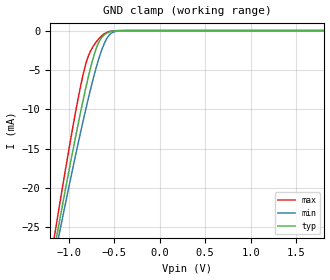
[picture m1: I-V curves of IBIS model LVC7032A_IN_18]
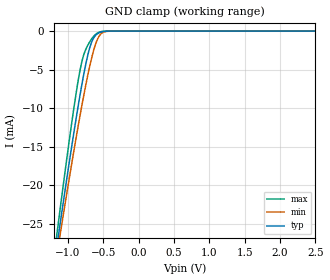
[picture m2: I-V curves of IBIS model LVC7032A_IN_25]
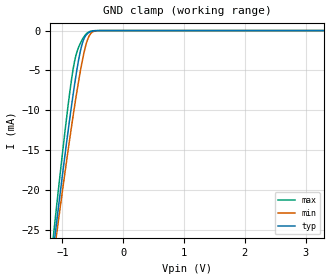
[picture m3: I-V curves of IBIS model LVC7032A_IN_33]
| TEXAS INSTRUMENTS INCORPORATED
| IBIS Model of SN74LVC7032A
| This file provides unique models under the [Model Selector] for each Vcc.
| For operation at a specific Vcc, select the appropriate model after each
| [Model Selector] keyword.
[IBIS Ver]   3.2
[Comment char]  |_char
[File Name]   sn74lvc7032aq1.ibs
[File Rev]   1
[Date]   October 2, 2023
[Source]   Data created from TI-SPICE simulations.
[Disclaimer] Property of Texas Instruments Incorporated.  Unauthorized
   reproduction and/or distribution is strictly prohibited.
   This product is protected under copyright law.
   Created  2023, (C) Copyright  2023, Texas Instruments
   Incorporated, All Rights Reserved
   UNLESS THERE IS A SIGNED, WRITTEN AGREEMENT TO THE
   CONTRARY, TEXAS INSTRUMENTS (TI) IS PROVIDING THE IBIS
   MODELS  AND WITHOUT ANY WARRANTY, EXPRESSED OR
   IMPLIED.  TI assumes no liability for:
   1) the accuracy of the IBIS models provided to your
   company;
   2) the proper functioning of these IBIS Models in your
   design or for any resulting applications; or
   3) infringement of patents, copyrights or intellectual
   property rights resulting from your use of these IBIS
   models.
   TI provides IBIS Models as a service to our customers.
   You and your company shall not distribute, sell or give
   these models to anyone else without prior written
   permission from TI.
   TI reserves the right to make changes to our products or
   to discontinue any semiconductor product or service
   without notice, and advises our customers to obtain the
   latest version of relevant information to verify, before
   placing orders, that the information being relied on is
   current.
   Please be aware that your receipt and use of the IBIS
   information provided shall serve as acceptance of these
   terms and conditions.  If you do not accept these terms,
   you should return or destroy the IBIS models and any
   other accompanying information immediately.
| Component LVC7032A_BQA 14-pin WQFN
[Component]   LVC7032A_BQA
[Manufacturer]   TI
[Package]   |14 WQFN - BQA package
|   typ   min   max
R_pkg   0.05   0.04   0.06
L_pkg   1.0nH   0.8nH   1.2nH
C_pkg   0.2pF   0.16pF   0.24pF
[Pin]   signal_name   model_name   R_pin   L_pin   C_pin
1   1A   LVC7032A_IN   NA   NA   NA
2   1B   LVC7032A_IN   NA   NA   NA
3   1Y   LVC7032A_OUT   NA   NA   NA
4   2A   LVC7032A_IN   NA   NA   NA
5   2B   LVC7032A_IN   NA   NA   NA
6   2Y   LVC7032A_OUT   NA   NA   NA
7   GND   GND   NA   NA   NA
8   3Y   LVC7032A_OUT   NA   NA   NA
9   3A   LVC7032A_IN   NA   NA   NA
10   3B   LVC7032A_IN   NA   NA   NA
11   4Y   LVC7032A_OUT   NA   NA   NA
12   4A   LVC7032A_IN   NA   NA   NA
13   4B   LVC7032A_IN   NA   NA   NA
14   VCC   POWER   NA   NA   NA
[Model Selector]   LVC7032A_IN
LVC7032A_IN_18   1.8 volt Vcc
LVC7032A_IN_25   2.5 volt Vcc
LVC7032A_IN_33   3.3 volt Vcc
| Model LVC7032A_OUT
[Model Selector]   LVC7032A_OUT
LVC7032A_OUT_18   1.8 volt Vcc
LVC7032A_OUT_25   2.5 volt Vcc
LVC7032A_OUT_33   3.3 volt Vcc
| Models and submodels in the file (6): LVC7032A_IN_18 (Input), LVC7032A_IN_25 (Input), LVC7032A_IN_33 (Input), LVC7032A_OUT_18 (Output), LVC7032A_OUT_25 (Output), LVC7032A_OUT_33 (Output)
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[Model]   LVC7032A_IN_18
Model_type  Input
Vinl=0.4
Vinh=0.85
| variable   typ   min   max
C_comp   2.66pF   2.19pF   3.17pF
[Temperature Range]   40   100   -40
| Ambient temperature   25   85   -40
[Voltage range]   1.8   1.65   1.95
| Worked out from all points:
|   GND clamp passes 1 mA (typ) near -0.64 V on its own axis
[GND Clamp]
| LVC7032A_IN_18
|   Voltage   I(typ)   I(min)   I(max)
-5.5V     -338.9mA   -314.3mA   -369mA
-1.16V    -28.09mA   -29.24mA   -26.56mA
-1.12V    -25.56mA   -26.92mA   -23.71mA
-1.085V   -23.36mA   -24.91mA   -21.25mA
-925mV    -13.65mA   -15.98mA   -10.52mA
-820mV    -7.797mA   -10.48mA   -4.654mA
-770mV    -5.293mA   -8.026mA   -2.891mA
-695mV    -2.253mA   -4.666mA   -1.432mA
-600mV    -473.7uA   -1.449mA   -358.4uA
-535mV    -136.2uA   -379.8uA   -78.5uA
-445mV    -16.2uA    -36.49uA   -4.833uA
1.8V      41.95pA    147.4pA    23.47pA
[Model]   LVC7032A_IN_25
Model_type  Input
Vinl=0.8
Vinh=1.2
| variable   typ   min   max
C_comp   2.58pF   2.03pF   3.24pF
[Temperature Range]   40   100   -40
| Ambient temperature   25   85   -40
[Voltage range]   2.5   2.3   2.7
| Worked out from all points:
|   GND clamp passes 1 mA (typ) near -0.64 V on its own axis
[GND Clamp]
| LVC7032A_IN_25
|   Voltage   I(typ)   I(min)   I(max)
-5.5V     -338.9mA   -314.3mA   -369mA
-1.17V    -28.73mA   -29.82mA   -27.27mA
-1.13V    -26.19mA   -27.5mA    -24.42mA
-1.095V   -23.98mA   -25.48mA   -21.95mA
-925mV    -13.65mA   -15.98mA   -10.52mA
-825mV    -8.06mA    -10.74mA   -4.88mA
-775mV    -5.531mA   -8.266mA   -3.027mA
-700mV    -2.416mA   -4.874mA   -1.51mA
-590mV    -396.4uA   -1.217mA   -293.2uA
-515mV    -88.16uA   -231.8uA   -44.89uA
-395mV    -4.232uA   -9.445uA   -775nA
2.5V      57.25pA    176.8pA    32.61pA
[Model]   LVC7032A_IN_33
Model_type  Input
Vinl=0.9
Vinh=1.5
| variable   typ   min   max
C_comp   2.50pF   1.92pF   3.16pF
[Temperature Range]   40   100   -40
| Ambient temperature   25   85   -40
[Voltage range]   3.3   3   3.6
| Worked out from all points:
|   GND clamp passes 1 mA (typ) near -0.64 V on its own axis
[GND Clamp]
| LVC7032A_IN_33
|   Voltage   I(typ)   I(min)   I(max)
-5.5V     -338.9mA   -314.3mA   -369mA
-1.14V    -26.82mA   -28.07mA   -25.13mA
-1.105V   -24.61mA   -26.05mA   -22.65mA
-1.075V   -22.73mA   -24.34mA   -20.55mA
-915mV    -13.07mA   -15.45mA   -9.893mA
-860mV    -9.954mA   -12.53mA   -6.658mA
-805mV    -7.019mA   -9.733mA   -4.027mA
-730mV    -3.528mA   -6.174mA   -2.02mA
-665mV    -1.428mA   -3.486mA   -1.009mA
-585mV    -362.1uA   -1.111mA   -263.9uA
-510mV    -78.77uA   -204.1uA   -38.82uA
3.3V      76.2pA     212.8pA    43.07pA
